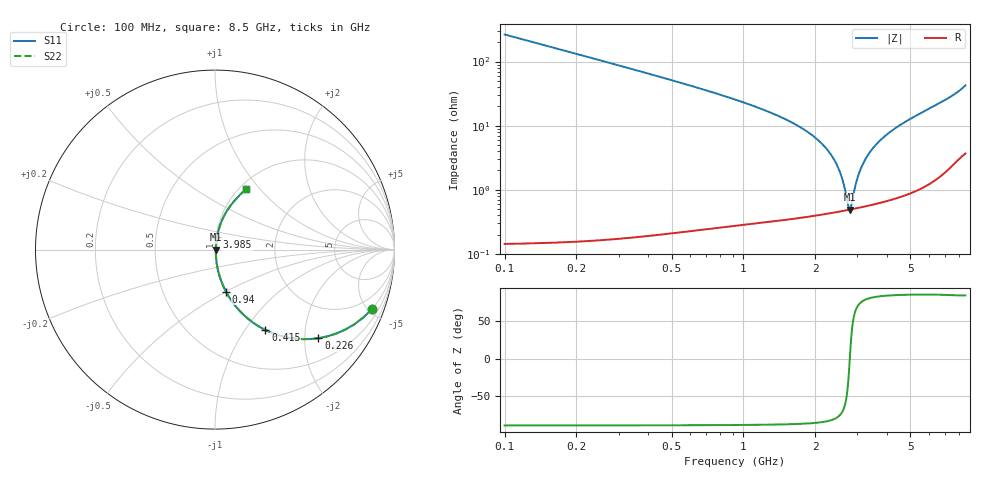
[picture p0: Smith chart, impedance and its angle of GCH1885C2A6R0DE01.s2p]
!Murata Part Number: GCH1885C2A6R0DE01
!These Parameters are Measured in Series Mode Connection
!Data Generated on Mar 13, 2026
!  o--ll--o
!Port1  Port2
!  o------o
!Operation Temp=25[degC], DC Bias Voltage=0[V]
!Freq. Start=100[MHz] Stop=9[GHz] 401[Steps]
# Hz S RI R 50
!Freq.(Hz) S11(Real) S11(Imag) S21(Real) S21(Imag) S12(Real) S12(Imag) S22(Real) S22(Imag)
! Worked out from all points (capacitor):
!   401 points, 100 MHz to 8.5 GHz, reference 50 ohm
!   read as one part in series: C = 6 pF near 142 MHz
!   lowest |Z| = 489 mohm at 2.788 GHz (marker M1)
!   series resonance near 2.789 GHz, so ESL is about 540 pH
!   S11 on the Smith chart (normalised r, x): 100 MHz: 1.00, -5.30; 226 MHz: 1.00, -2.33; 415 MHz: 1.00, -1.25; 940 MHz: 1.01, -0.50; 3.985 GHz: 1.01, +0.14; 8.5 GHz: 1.07, +0.85
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1e8  0.8751 -0.3303  0.1249 0.3303  0.1249 0.3303  0.8751 -0.3303
2.26e8  0.5759 -0.4935  0.4241 0.4935  0.4241 0.4935  0.5759 -0.4935
3.1e8  0.4166 -0.492  0.5834 0.492  0.5834 0.492  0.4166 -0.492
4.15e8  0.2812 -0.4481  0.7188 0.4481  0.7188 0.4481  0.2812 -0.4481
6.25e8  0.141 -0.3451  0.859 0.3451  0.859 0.3451  0.141 -0.3451
9.4e8  0.0611 -0.234  0.9389 0.234  0.9389 0.234  0.0611 -0.234
1.507e9  0.0186 -0.1221  0.9814 0.1221  0.9814 0.1221  0.0186 -0.1221
2.011e9  0.00793 -0.0629  0.9921 0.0629  0.9921 0.0629  0.00793 -0.0629
2.347e9  0.00542 -0.033  0.9946 0.033  0.9946 0.033  0.00542 -0.033
2.557e9  0.00485 -0.0166  0.9951 0.0166  0.9951 0.0166  0.00485 -0.0166
2.746e9  0.00482 -0.00295  0.9952 0.00295  0.9952 0.00295  0.00482 -0.00295
2.788e9  0.00487 -4.25e-05  0.9951 4.25e-05  0.9951 4.25e-05  0.00487 -4.25e-05
2.83e9  0.00493 0.00282  0.9951 -0.00282  0.9951 -0.00282  0.00493 0.00282
2.914e9  0.0051 0.00843  0.9949 -0.00843  0.9949 -0.00843  0.0051 0.00843
3.061e9  0.00555 0.0179  0.9945 -0.0179  0.9945 -0.0179  0.00555 0.0179
3.271e9  0.00647 0.0309  0.9935 -0.0309  0.9935 -0.0309  0.00647 0.0309
3.565e9  0.00826 0.048  0.9917 -0.048  0.9917 -0.048  0.00826 0.048
3.985e9  0.0117 0.0711  0.9883 -0.0711  0.9883 -0.0711  0.0117 0.0711
4.3e9  0.015 0.0876  0.985 -0.0876  0.985 -0.0876  0.015 0.0876
5.707e9  0.0371 0.159  0.9629 -0.159  0.9629 -0.159  0.0371 0.159
7.114e9  0.0796 0.2355  0.9204 -0.2355  0.9204 -0.2355  0.0796 0.2355
8.5e9  0.1737 0.3381  0.8263 -0.3381  0.8263 -0.3381  0.1737 0.3381
